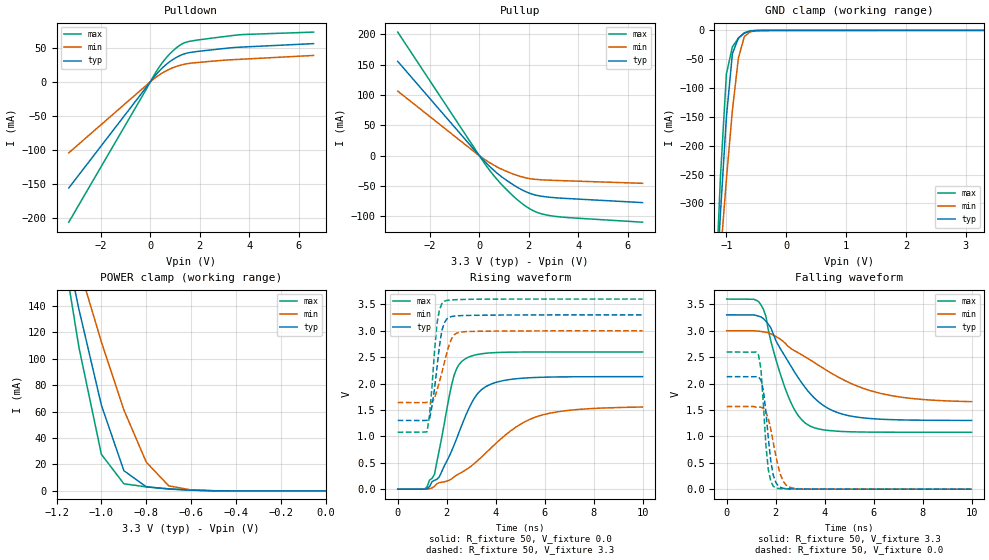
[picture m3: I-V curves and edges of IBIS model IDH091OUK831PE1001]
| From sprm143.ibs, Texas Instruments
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[Model]   IDH091OUK831PE1001
| I/O with pulldown
Model_type   I/O
Vinh = 2.00
Vinl = 0.80
Enable   Active-Low
Polarity   Non-Inverting
| signals   A, GZ, Y
Vmeas = 1.5
|   typ   min   max
C_comp   1.4592p   1.4336p   1.5063p
|   typ   min   max
[Temperature Range]   25   -40   125
|   typ   min   max
[Voltage Range]   3.30V   3.00V   3.60V
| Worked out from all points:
|   slope of the pulldown table from 0 to 0.495 V, typ, clamps not added: 24 ohm
|   slope of the pullup table from 0 to 0.495 V, typ, clamps not added: 23.8 ohm
|   GND clamp passes 1 mA (typ) near -0.60 V on its own axis
|   POWER clamp passes 1 mA (typ) near -0.65 V on its own axis
|   rising waveform, R_fixture 50, V_fixture 0.0: 20-80 % time 1.22ns typ, 2.49ns min, 659ps max; typ from 0 V to 2.13 V
|   falling waveform, R_fixture 50, V_fixture 3.3: 20-80 % time 1.7ns typ, 3.03ns min, 1.01ns max; typ from 3.3 V to 1.3 V
|   rising waveform, R_fixture 50, V_fixture 3.3: 20-80 % time 327ps typ, 469ps min, 262ps max; typ from 1.3 V to 3.3 V
|   falling waveform, R_fixture 50, V_fixture 0.0: 20-80 % time 301ps typ, 433ps min, 240ps max; typ from 2.13 V to 0 V
[Pulldown]
|   Voltage   I(typ)   I(min)   I(max)
-3.3V     -155.6mA   -104.1mA   -205.6mA
200mV     9.243mA    5.866mA    12.7mA
600mV     24.13mA    15.28mA    33.3mA
800mV     29.87mA    18.87mA    41.37mA
1.1V      36.63mA    23.02mA    51.08mA
1.3V      39.97mA    25.04mA    55.82mA
1.6V      42.83mA    27mA       59.29mA
3.5V      50.44mA    32.65mA    68.4mA
6.6V      55.87mA    38.54mA    72.75mA
[GND_clamp]
|   Voltage   I(typ)   I(min)   I(max)
-3.3V     -4.929A    -3.713A    -6.403A
-1.2V     -505.8mA   -530.1mA   -497.5mA
-1.1V     -317.7mA   -390.9mA   -254.9mA
-1V       -149.9mA   -258.2mA   -75.34mA
-900mV    -40.43mA   -138.4mA   -28.43mA
-800mV    -13.11mA   -48.15mA   -13.6mA
-700mV    -4.74mA    -10.34mA   -4.028mA
-600mV    -956.8uA   -2.434mA   -531.5uA
-400mV    -40.57uA   -72.23uA   -55.69uA
3.3V      100.3uA    53.87uA    176.6uA
[Pullup]
|   Voltage   I(typ)   I(min)   I(max)
-3.3V     155.5mA    106.5mA    203.9mA
-200mV    9.306mA    6.233mA    12.42mA
300mV     -13.07mA   -8.546mA   -17.75mA
600mV     -24.68mA   -16mA      -33.65mA
900mV     -34.78mA   -22.33mA   -47.64mA
1.4V      -48.81mA   -30.78mA   -67.77mA
1.7V      -55.9mA    -34.78mA   -78.19mA
2V        -61.53mA   -37.68mA   -86.71mA
2.3V      -65.31mA   -39.22mA   -93.01mA
2.9V      -68.83mA   -40.61mA   -99.22mA
3.7V      -71.03mA   -41.73mA   -102.5mA
6.6V      -77.46mA   -45.65mA   -109.8mA
[POWER_clamp]
|   Voltage   I(typ)   I(min)   I(max)
-3.3V     2.11A      1.592A     2.739A
-1.2V     217.8mA    229.1mA    213mA
-1.1V     137.1mA    169.4mA    108.4mA
-1V       64.78mA    112.6mA    27.62mA
-900mV    15.3mA     61.21mA    5.429mA
-800mV    3.096mA    21.71mA    3.058mA
-700mV    1.437mA    3.856mA    1.578mA
-600mV    596.4uA    717.5uA    553.1uA
-500mV    141uA      150.6uA    81.58uA
0V        0A         0A         0A
[Ramp]
|   I(typ)   I(min)   I(max)
dV/dt_r   1.278/1.217n   0.933/2.484n   1.559/0.655n
dV/dt_f   1.199/1.705n   0.806/3.029n   1.513/1.012n
[Rising Waveform]
R_fixture = 50
V_fixture = 0.0
|  pu_on
|  TIME   V(typ)   V(min)   V(max)
0s        5nV        19nV       4nV
1.1ns     -60.64uV   -120.3uV   2.128mV
1.5ns     166.8mV    52.5mV     278.8mV
1.7ns     232.6mV    123.4mV    746.5mV
2.3ns     833.1mV    231.3mV    2.151V
2.8ns     1.419V     370.9mV    2.478V
3.2ns     1.771V     513.9mV    2.545V
3.6ns     1.942V     686.2mV    2.574V
5.6ns     2.114V     1.361V     2.597V
10ns      2.131V     1.555V     2.598V
[Falling Waveform]
R_fixture = 50
V_fixture = 3.3
V_fixture_min = 3.0
V_fixture_max = 3.6
|  pd_on
|  TIME   V(typ)   V(min)   V(max)
0s        3.3V       3V         3.6V
1.4ns     3.262V     2.987V     3.491V
1.6ns     3.181V     2.973V     3.276V
1.8ns     3.058V     2.943V     2.811V
2.5ns     2.425V     2.708V     1.773V
2.9ns     2.126V     2.588V     1.407V
3.4ns     1.815V     2.45V      1.197V
5.1ns     1.381V     1.998V     1.086V
7ns       1.313V     1.751V     1.078V
10ns      1.302V     1.657V     1.078V
[Rising Waveform]
R_fixture = 50
V_fixture = 3.3
V_fixture_min = 3.0
V_fixture_max = 3.6
|  pd_off
|  TIME   V(typ)   V(min)   V(max)
0s        1.301V     1.64V      1.078V
1.2ns     1.306V     1.644V     1.087V
1.3ns     1.332V     1.648V     1.413V
1.4ns     1.572V     1.648V     1.94V
1.6ns     2.287V     1.867V     3.124V
1.8ns     2.998V     2.202V     3.511V
1.9ns     3.149V     2.391V     3.557V
2.2ns     3.269V     2.85V      3.584V
2.6ns     3.286V     2.976V     3.592V
10ns      3.3V       3V         3.6V
[Falling Waveform]
R_fixture = 50
V_fixture = 0.0
|  pu_off
|  TIME   V(typ)   V(min)   V(max)
0s        2.131V     1.565V     2.598V
1.3ns     2.126V     1.555V     2.541V
1.4ns     2.062V     1.552V     2.267V
1.5ns     1.87V      1.532V     1.599V
1.7ns     967.9mV    1.337V     367.8mV
1.8ns     541.4mV    1.136V     154.3mV
2ns       133.1mV    645mV      22.93mV
2.3ns     18.01mV    159.7mV    6.512mV
2.7ns     5.598mV    19.92mV    3.111mV
10ns      2.535uV    61.82uV    1.544uV
